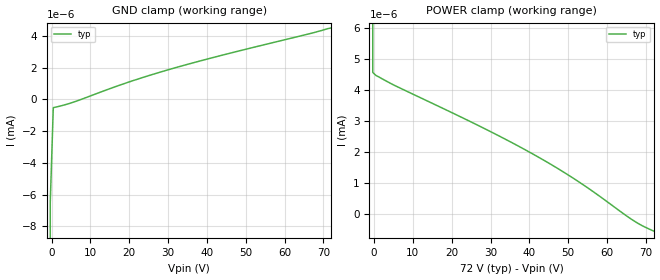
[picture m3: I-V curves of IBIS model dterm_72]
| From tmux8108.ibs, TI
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| dterm_72
[Model]   dterm_72
Model_type   Terminator
|   typ   min   max
C_comp   1.008417e-11   NA   NA
[Voltage Range]   72   NA   NA
[Temperature Range]   27   NA   NA
[Power Clamp Reference]   72   NA   NA
[GND Clamp Reference]   0   NA   NA
[GND Clamp]
|   Voltage   I(typ)   I(min)   I(max)
-5V       -4.511A    NA         NA
-1.111V   -72.69mA   NA         NA
-333.3mV  -6.477nA   NA         NA
444.4mV   -524.1pA   NA         NA
5.111V    -218.2pA   NA         NA
19.11V    1.024nA    NA         NA
30.78V    1.913nA    NA         NA
43.22V    2.735nA    NA         NA
72V       4.494nA    NA         NA
[POWER Clamp]
|   Voltage   I(typ)   I(min)   I(max)
-5V       1.488A     NA         NA
-1.111V   52.26mA    NA         NA
-333.3mV  4.568nA    NA         NA
444.4mV   4.474nA    NA         NA
5.111V    4.16nA     NA         NA
28.44V    2.756nA    NA         NA
40.89V    1.936nA    NA         NA
52.56V    1.052nA    NA         NA
66.56V    -191.2pA   NA         NA
68.89V    -365.1pA   NA         NA
72V       -549pA     NA         NA
